PROGRAM p08_stevnik
VAR
	stevnik: CTUD;
	S0: BOOL;
	S1: BOOL;
	S2: BOOL;
	S3: BOOL;
	vrednost: WORD;
END_VAR

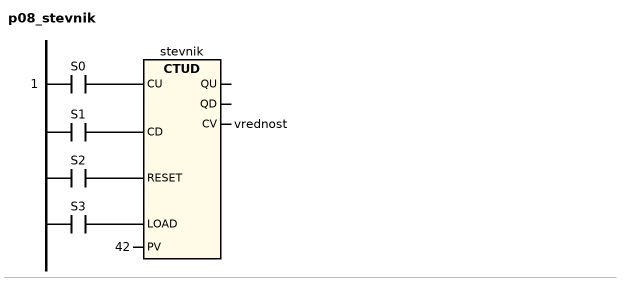
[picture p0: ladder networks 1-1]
// NETWORK 1
stevnik(CU := S0, CD := S1, RESET := S2, LOAD := S3, PV := 42, CV => vrednost); // CTUD

END_PROGRAM
